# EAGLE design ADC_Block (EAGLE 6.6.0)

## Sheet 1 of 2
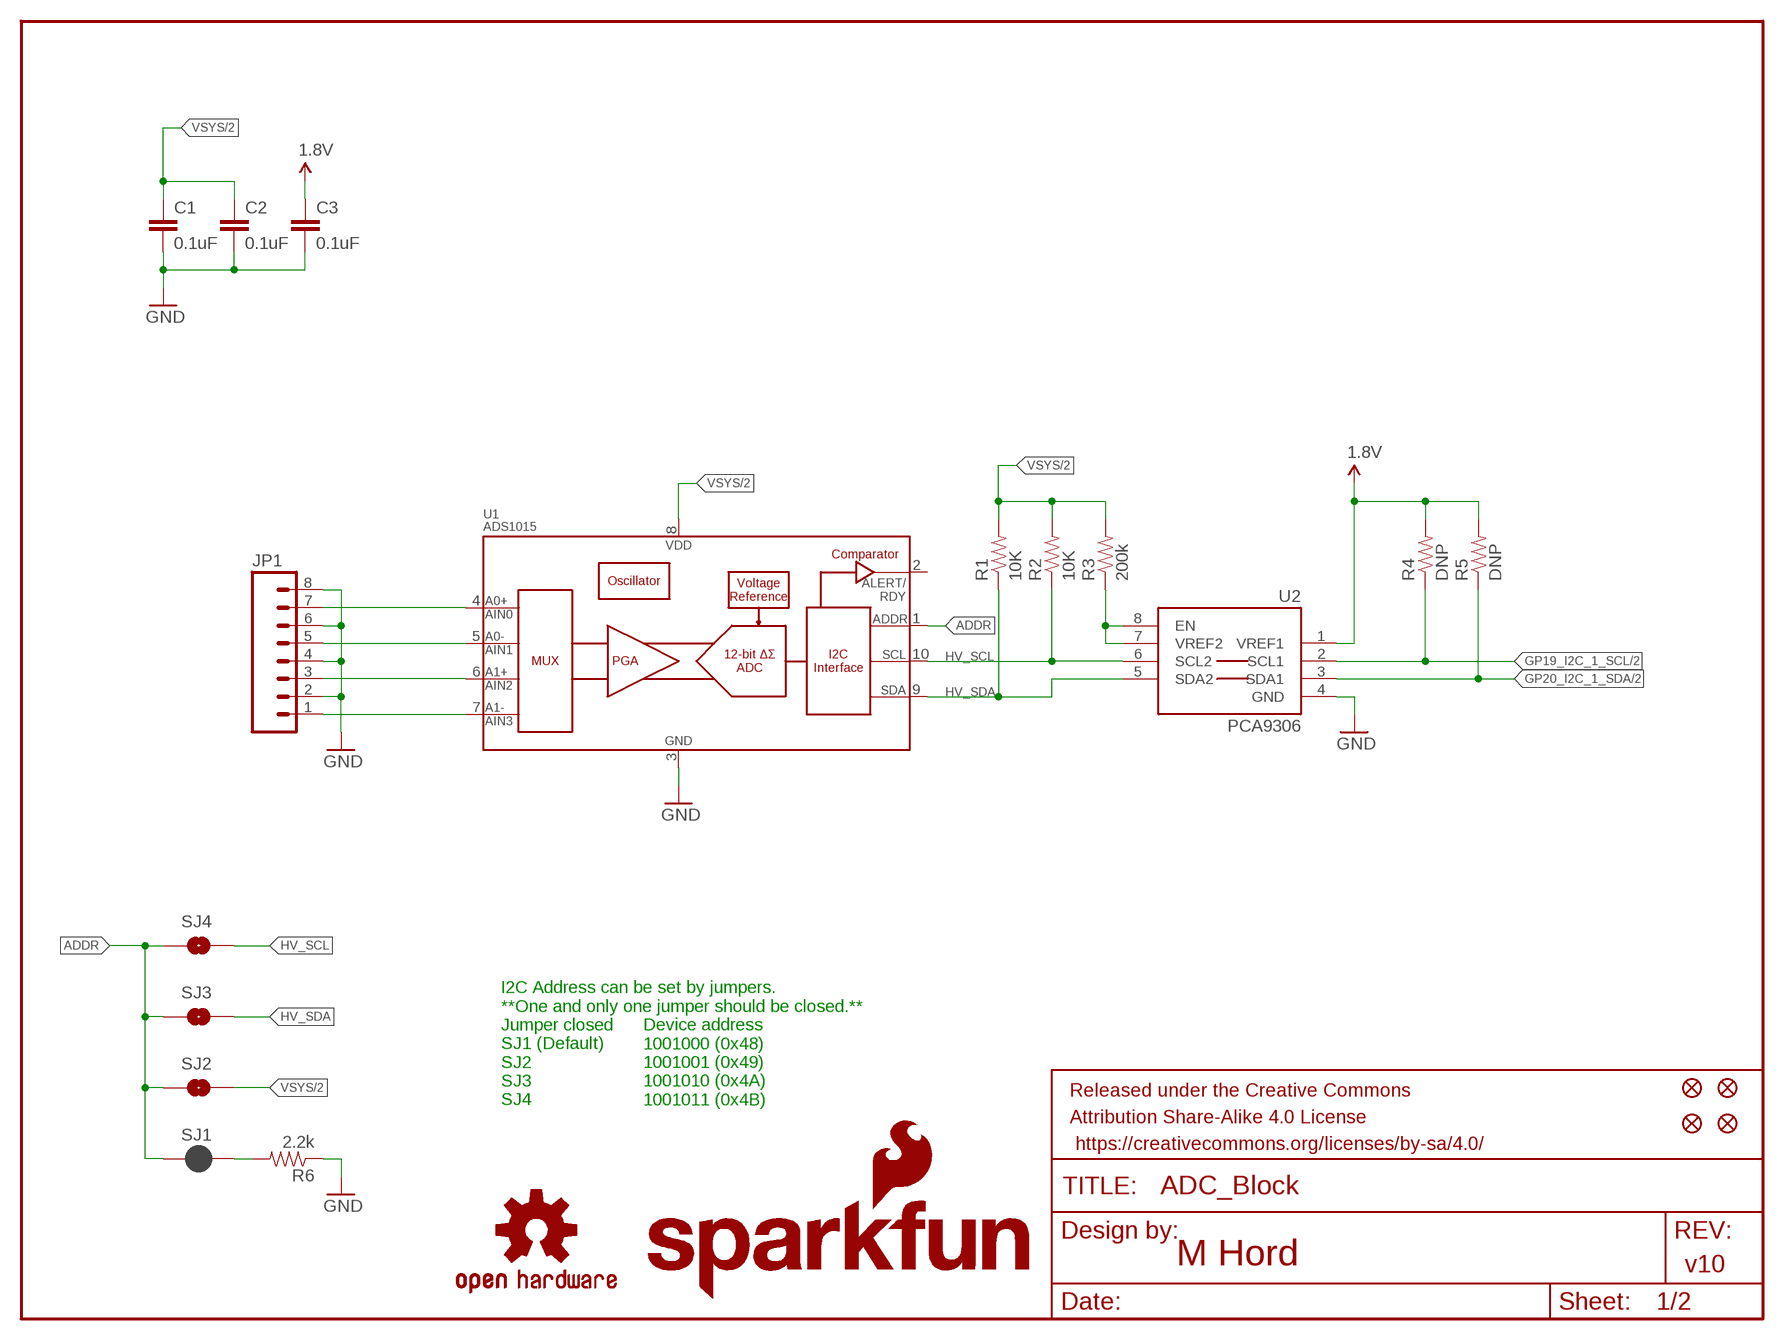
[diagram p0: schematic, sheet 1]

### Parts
C1  0.1uF  0.1UF-25V(+80/-20%)(0603)  [0603-CAP]
C2  0.1uF  0.1UF-25V(+80/-20%)(0603)  [0603-CAP]
C3  0.1uF  0.1UF-25V(+80/-20%)(0603)  [0603-CAP]
FID1  FIDUCIAL1X2  [FIDUCIAL-1X2]
FID2  FIDUCIAL1X2  [FIDUCIAL-1X2]
FID3  FIDUCIAL1X2  [FIDUCIAL-1X2]
FID4  FIDUCIAL1X2  [FIDUCIAL-1X2]
FRAME1  FRAME-LETTER  [CREATIVE_COMMONS]
JP1  M081X08  [1X08]
LOGO1  SFE_LOGO_NAME_FLAME.1_INCH  [SFE_LOGO_NAME_FLAME_.1]
LOGO2  OSHW-LOGOS  [OSHW-LOGO-S]
LOGO3  SFE_LOGO_NAME_FLAME.1_INCH  [SFE_LOGO_NAME_FLAME_.1]
LOGO4  OSHW-LOGOS  [OSHW-LOGO-S]
R1  10K  10KOHM1/10W1%(0603)0603  [0603-RES]
R2  10K  10KOHM1/10W1%(0603)0603  [0603-RES]
R3  200k  200KOHM1/10W1%(0603)200K  [0603-RES]
R4  DNP  2.2KOHM1/10W1%(0603)  [0603-RES]
R5  DNP  2.2KOHM1/10W1%(0603)  [0603-RES]
R6  2.2k  2.2KOHM1/10W1%(0603)  [0603-RES]
SJ1  JUMPER-PAD-2-NC_BY_PASTE  [PAD-JUMPER-2-NC_BY_PASTE_YES_SILK]
SJ2  JUMPER-PAD-2-NOYES_SILK  [PAD-JUMPER-2-NO_YES_SILK]
SJ3  JUMPER-PAD-2-NOYES_SILK  [PAD-JUMPER-2-NO_YES_SILK]
SJ4  JUMPER-PAD-2-NOYES_SILK  [PAD-JUMPER-2-NO_YES_SILK]
U1  ADS1015  [MSOP10]
U2  PCA9306  PCA9306PCA9306DC-1:1  [PCA9306DC-1:1]

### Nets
1.8V: C3.1 R4.2 R5.2 U2.1(VREF1) ; also sheet 2
A0+/AIN0: JP1.7 U1.4(AIN0)
A0-/AIN1: JP1.5 U1.5(AIN1)
A1+/AIN2: JP1.3 U1.6(AIN2)
A1-/AIN3: JP1.1 U1.7(AIN3)
ADDR: SJ1.1 SJ2.1 SJ3.1 SJ4.1 U1.1(ADDR)
GND: C1.2 C2.2 C3.2 JP1.2 JP1.4 JP1.6 JP1.8 R6.1 U1.3(VSS) U2.4(GND) ; also sheet 2
GP19_I2C_1_SCL: R4.1 U2.2(SCL1) ; also sheet 2
GP20_I2C_1_SDA: R5.1 U2.3(SDA1) ; also sheet 2
HV_SCL: R2.1 SJ4.2 U1.10(SCL) U2.6(SCL2)
HV_SDA: R1.1 SJ3.2 U1.9(SDA) U2.5(SDA2)
N$1: R3.1 U2.7(VREF2) U2.8(EN)
N$3: R6.2 SJ1.2
VSYS: C1.1 C2.1 R1.2 R2.2 R3.2 SJ2.2 U1.8(VDD) ; also sheet 2
Unconnected: U1.2(ALERT/RDY)

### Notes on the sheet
- I2C Address can be set by jumpers.
  **One and only one jumper should be closed.**
  Jumper closed
  SJ1 (Default)
  SJ2
  SJ3
  SJ4
- Device address
  1001000 (0x48)
  1001001 (0x49)
  1001010 (0x4A)
  1001011 (0x4B)
- M Hord
- v10

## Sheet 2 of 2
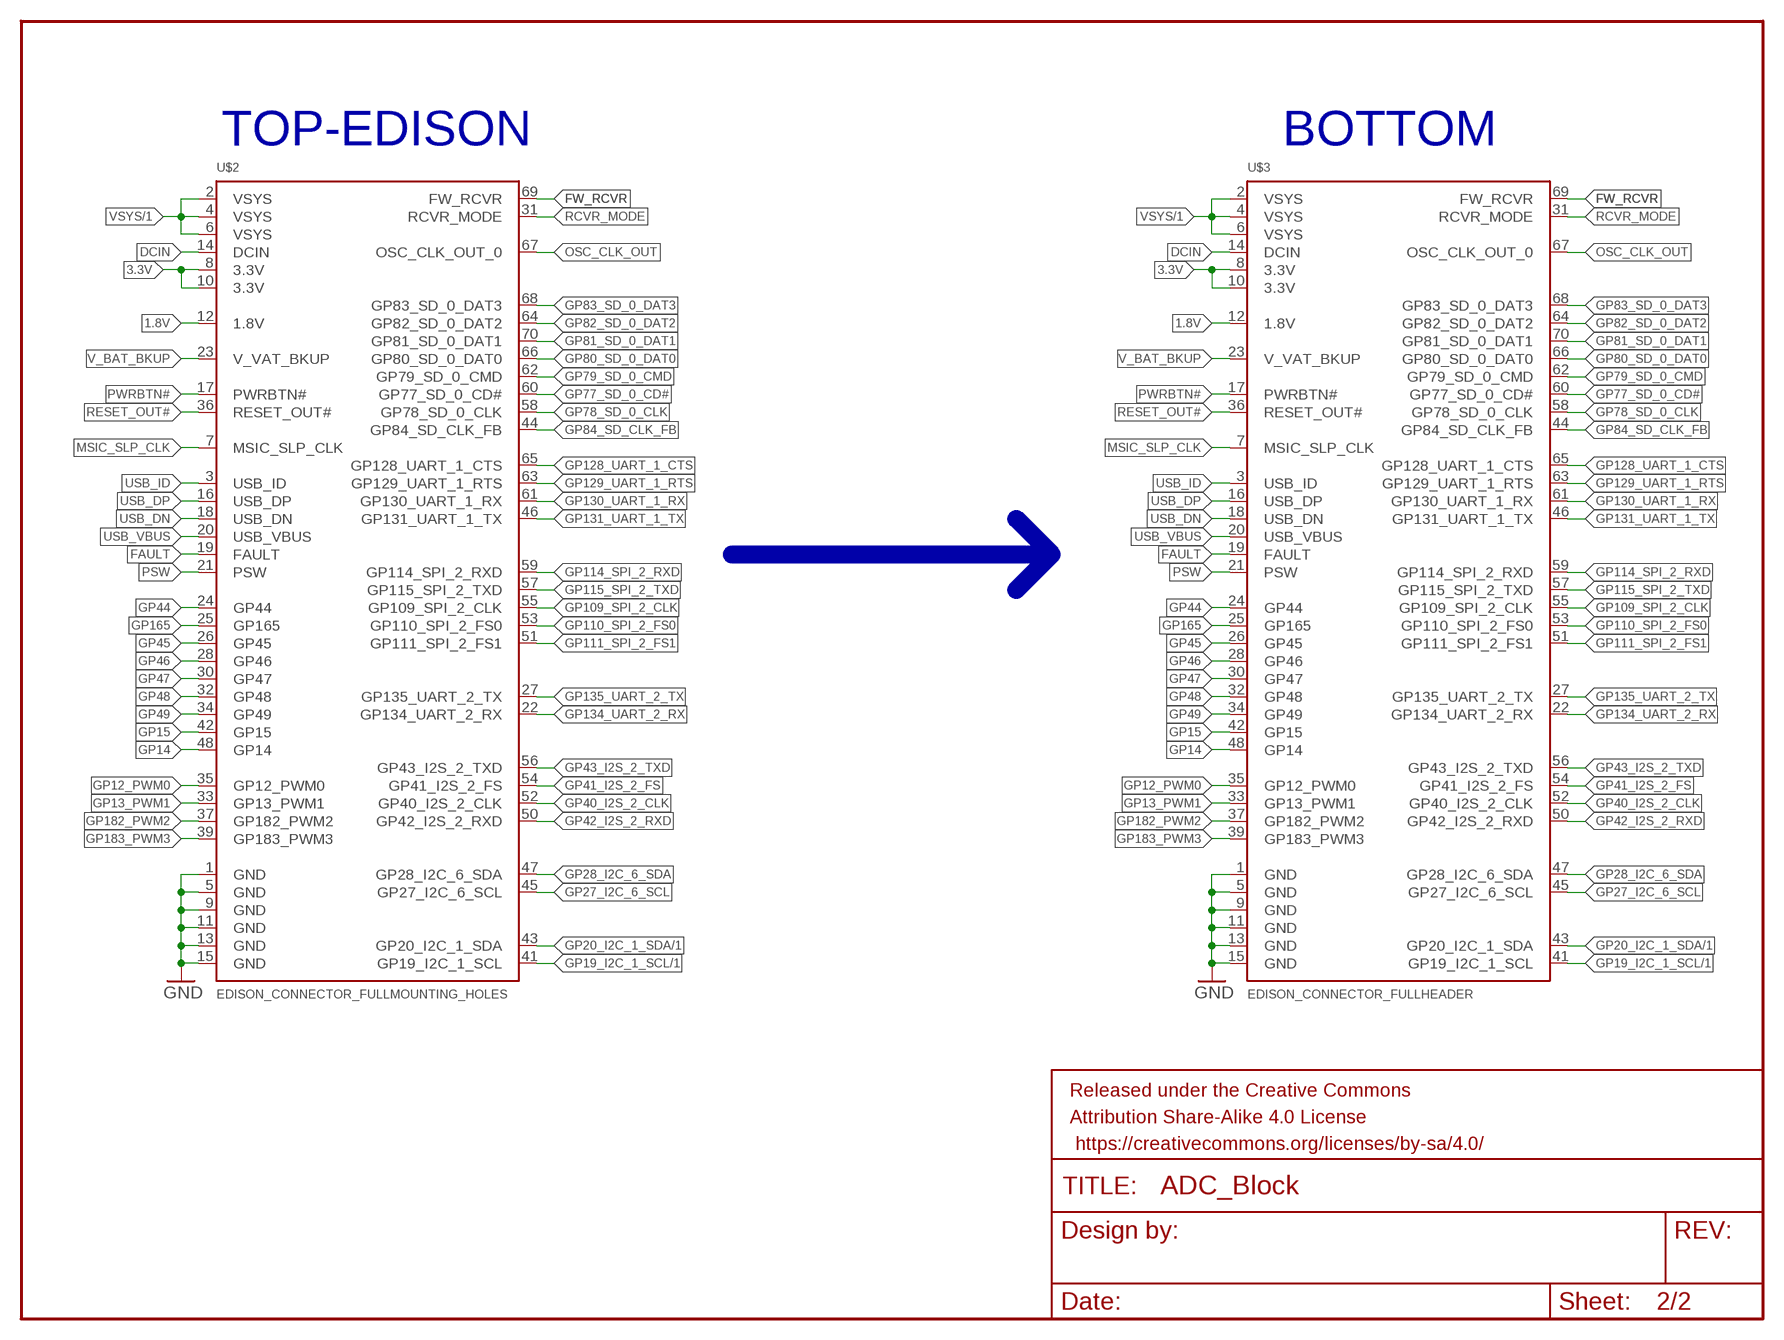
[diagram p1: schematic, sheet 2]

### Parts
FRAME2  FRAME-LETTER  [CREATIVE_COMMONS]
U$2  EDISON_CONNECTOR_FULLMOUNTING_HOLES  [EDISON_DAUGHTER]
U$3  EDISON_CONNECTOR_FULLHEADER  [DF40C-70DP-0.4(51)]

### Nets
1.8V: U$2.12(1.8V) U$3.12(1.8V) ; also sheet 1
3.3V: U$2.8(3.3V) U$2.10(3.3V) U$3.8(3.3V) U$3.10(3.3V)
DCIN: U$2.14(DCIN) U$3.14(DCIN)
FAULT: U$2.19(FAULT) U$3.19(FAULT)
FW_RCVR: U$2.69(FW_RCVR) U$3.69(FW_RCVR)
GND: U$2.1(GND) U$2.5(GND) U$2.9(GND) U$2.11(GND) U$2.13(GND) U$2.15(GND) U$3.1(GND) U$3.5(GND) U$3.9(GND) U$3.11(GND) U$3.13(GND) U$3.15(GND) ; also sheet 1
GP12_PWM0: U$2.35(GP12_PWM0) U$3.35(GP12_PWM0)
GP13_PWM1: U$2.33(GP13_PWM1) U$3.33(GP13_PWM1)
GP14: U$2.48(GP14) U$3.48(GP14)
GP15: U$2.42(GP15) U$3.42(GP15)
GP19_I2C_1_SCL: U$2.41(GP19_I2C_1_SCL) U$3.41(GP19_I2C_1_SCL) ; also sheet 1
GP20_I2C_1_SDA: U$2.43(GP20_I2C_1_SDA) U$3.43(GP20_I2C_1_SDA) ; also sheet 1
GP27_I2C_6_SCL: U$2.45(GP27_I2C_6_SCL) U$3.45(GP27_I2C_6_SCL)
GP28_I2C_6_SDA: U$2.47(GP28_I2C_6_SDA) U$3.47(GP28_I2C_6_SDA)
GP40_I2S_2_CLK: U$2.52(GP40_I2S_2_CLK) U$3.52(GP40_I2S_2_CLK)
GP41_I2S_2_FS: U$2.54(GP41_I2S_2_FS) U$3.54(GP41_I2S_2_FS)
GP42_I2S_2_RXD: U$2.50(GP42_I2S_2_RXD) U$3.50(GP42_I2S_2_RXD)
GP43_I2S_2_TXD: U$2.56(GP43_I2S_2_TXD) U$3.56(GP43_I2S_2_TXD)
GP44: U$2.24(GP44) U$3.24(GP44)
GP45: U$2.26(GP45) U$3.26(GP45)
GP46: U$2.28(GP46) U$3.28(GP46)
GP47: U$2.30(GP47) U$3.30(GP47)
GP48: U$2.32(GP48) U$3.32(GP48)
GP49: U$2.34(GP49) U$3.34(GP49)
GP77_SD_0_CD#: U$2.60(GP77_SD_0_CD#) U$3.60(GP77_SD_0_CD#)
GP78_SD_0_CLK: U$2.58(GP78_SD_0_CLK) U$3.58(GP78_SD_0_CLK)
GP79_SD_0_CMD: U$2.62(GP79_SD_0_CMD) U$3.62(GP79_SD_0_CMD)
GP80_SD_0_DAT0: U$2.66(GP80_SD_0_DAT0) U$3.66(GP80_SD_0_DAT0)
GP81_SD_0_DAT1: U$2.70(GP81_SD_0_DAT1) U$3.70(GP81_SD_0_DAT1)
GP82_SD_0_DAT2: U$2.64(GP82_SD_0_DAT2) U$3.64(GP82_SD_0_DAT2)
GP83_SD_0_DAT3: U$2.68(GP83_SD_0_DAT3) U$3.68(GP83_SD_0_DAT3)
GP84_SD_CLK_FB: U$2.44(GP84_SD_CLK_FB) U$3.44(GP84_SD_CLK_FB)
GP109_SPI_2_CLK: U$2.55(GP109_SPI_2_CLK) U$3.55(GP109_SPI_2_CLK)
GP110_SPI_2_FS0: U$2.53(GP110_SPI_2_FS0) U$3.53(GP110_SPI_2_FS0)
GP111_SPI_2_FS1: U$2.51(GP111_SPI_2_FS1) U$3.51(GP111_SPI_2_FS1)
GP114_SPI_2_RXD: U$2.59(GP114_SPI_2_RXD) U$3.59(GP114_SPI_2_RXD)
GP115_SPI_2_TXD: U$2.57(GP115_SPI_2_TXD) U$3.57(GP115_SPI_2_TXD)
GP128_UART_1_CTS: U$2.65(GP128_UART_1_CTS) U$3.65(GP128_UART_1_CTS)
GP129_UART_1_RTS: U$2.63(GP129_UART_1_RTS) U$3.63(GP129_UART_1_RTS)
GP130_UART_1_RX: U$2.61(GP130_UART_1_RX) U$3.61(GP130_UART_1_RX)
GP131_UART_1_TX: U$2.46(GP131_UART_1_TX) U$3.46(GP131_UART_1_TX)
GP134_UART_2_RX: U$2.22(GP134_UART_2_RX) U$3.22(GP134_UART_2_RX)
GP135_UART_2_TX: U$2.27(GP135_UART_2_TX) U$3.27(GP135_UART_2_TX)
GP165: U$2.25(GP165) U$3.25(GP165)
GP182_PWM2: U$2.37(GP182_PWM2) U$3.37(GP182_PWM2)
GP183_PWM3: U$2.39(GP183_PWM3) U$3.39(GP183_PWM3)
MSIC_SLP_CLK: U$2.7(MSIC_SLP_CLK) U$3.7(MSIC_SLP_CLK)
OSC_CLK_OUT: U$2.67(OSC_CLK_OUT_0) U$3.67(OSC_CLK_OUT_0)
PSW: U$2.21(PSW) U$3.21(PSW)
PWRBTN#: U$2.17(PWRBTN#) U$3.17(PWRBTN#)
RCVR_MODE: U$2.31(RCVR_MODE) U$3.31(RCVR_MODE)
RESET_OUT#: U$2.36(RESET_OUT#) U$3.36(RESET_OUT#)
USB_DN: U$2.18(USB_DN) U$3.18(USB_DN)
USB_DP: U$2.16(USB_DP) U$3.16(USB_DP)
USB_ID: U$2.3(USB_ID) U$3.3(USB_ID)
USB_VBUS: U$2.20(USB_VBUS) U$3.20(USB_VBUS)
V_BAT_BKUP: U$2.23(V_VAT_BKUP) U$3.23(V_VAT_BKUP)
VSYS: U$2.2(VSYS) U$2.4(VSYS) U$2.6(VSYS) U$3.2(VSYS) U$3.4(VSYS) U$3.6(VSYS) ; also sheet 1

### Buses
B$1

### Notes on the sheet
- TOP-EDISON | BOTTOM

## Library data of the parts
C1-C3 = SparkFun-Capacitors:0.1UF-25V(+80/-20%)(0603): CAP-00810; PROD_ID: CAP-00810
FID1-FID4 = SparkFun-Aesthetics:FIDUCIAL: Fiducial Alignment Points
FRAME1 FRAME2 = SparkFun-Aesthetics:FRAME-LETTER: Schematic Frame
JP1 = SparkFun-Connectors:M08: Header 8 Standard 8-pin 0.1" header. Use with straight break away headers (SKU : PRT-00116), right angle break away headers (PRT-00553), swiss pins (PRT-00743), machine pins (PRT-00117), and female headers (PRT-00115).
LOGO1 LOGO3 = SparkFun-Aesthetics:SFE_LOGO_NAME_FLAME: SFE Logo, name and flame
LOGO2 LOGO4 = SparkFun-Aesthetics:OSHW-LOGO: Open Source Hardware Logo This logo indicates the piece of hardware it is found on incorporates a OSHW license and/or adheres to the definition of open source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
R1 R2 = SparkFun-Resistors:10KOHM1/10W1%(0603): RES-00824; PROD_ID: RES-00824
R3 = SparkFun-Resistors:200KOHM1/10W1%(0603): RES-09385; PROD_ID: RES-09385
R4 R5 = SparkFun-Resistors:2.2KOHM1/10W1%(0603): RES-08272; PROD_ID: RES-08272; VALUE: 2.2k
R6 = SparkFun-Resistors:2.2KOHM1/10W1%(0603): RES-08272; PROD_ID: RES-08272
SJ1 = SparkFun-Passives:JUMPER-PAD-2-NC_BY_PASTE
SJ2-SJ4 = SparkFun-Passives:JUMPER-PAD-2-NO
U1 = SparkFun-AnalogIC:ADS1015: 12-Bit Del-Sig ADC Four single-ended inputs or two differential inputs Internal PGA I2C interface 2.0-5.5V; PROD_ID: IC-12239
U2 = SparkFun-DigitalIC:PCA9306: Bidirectional I2C level shifter. NOT compatible with all available part number pinout schemes- DOUBLE CHECK!!!; PROD_ID: IC-10023
U$2 U$3 = Edison:EDISON_CONNECTOR_FULL

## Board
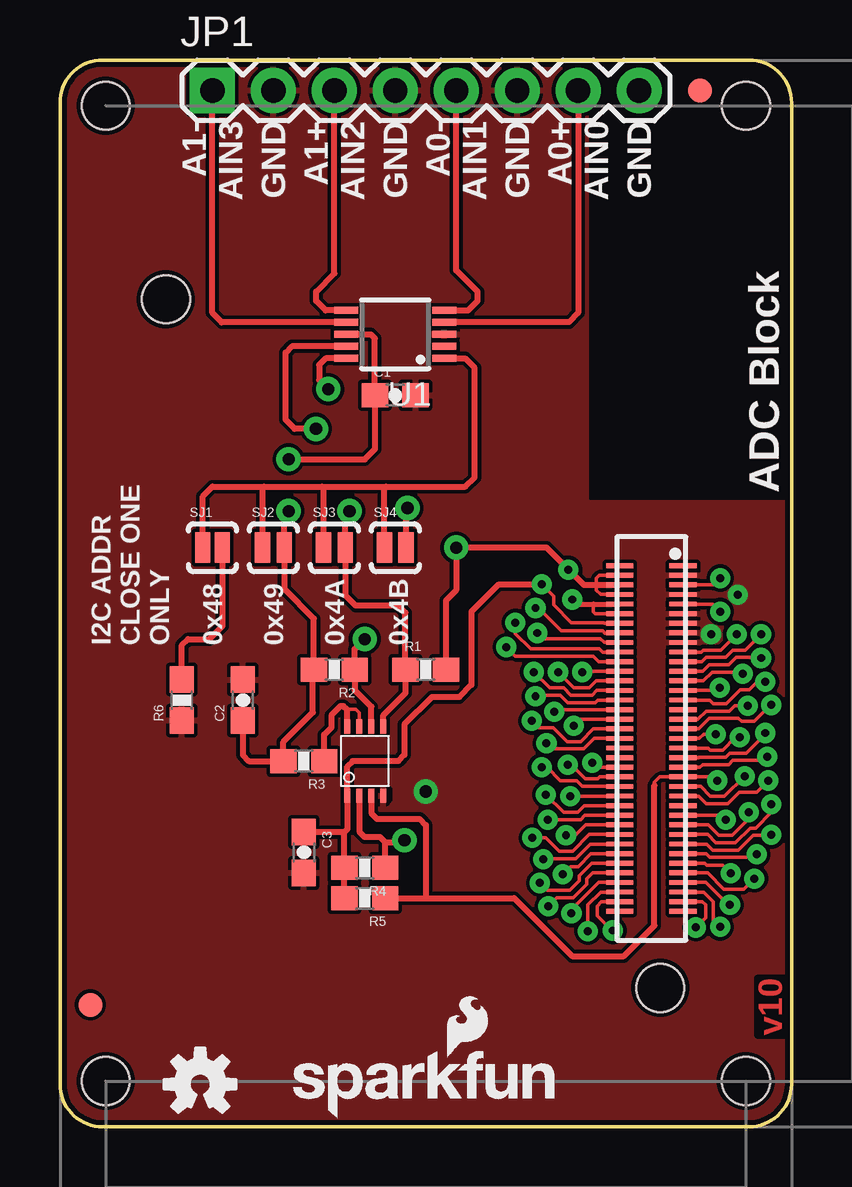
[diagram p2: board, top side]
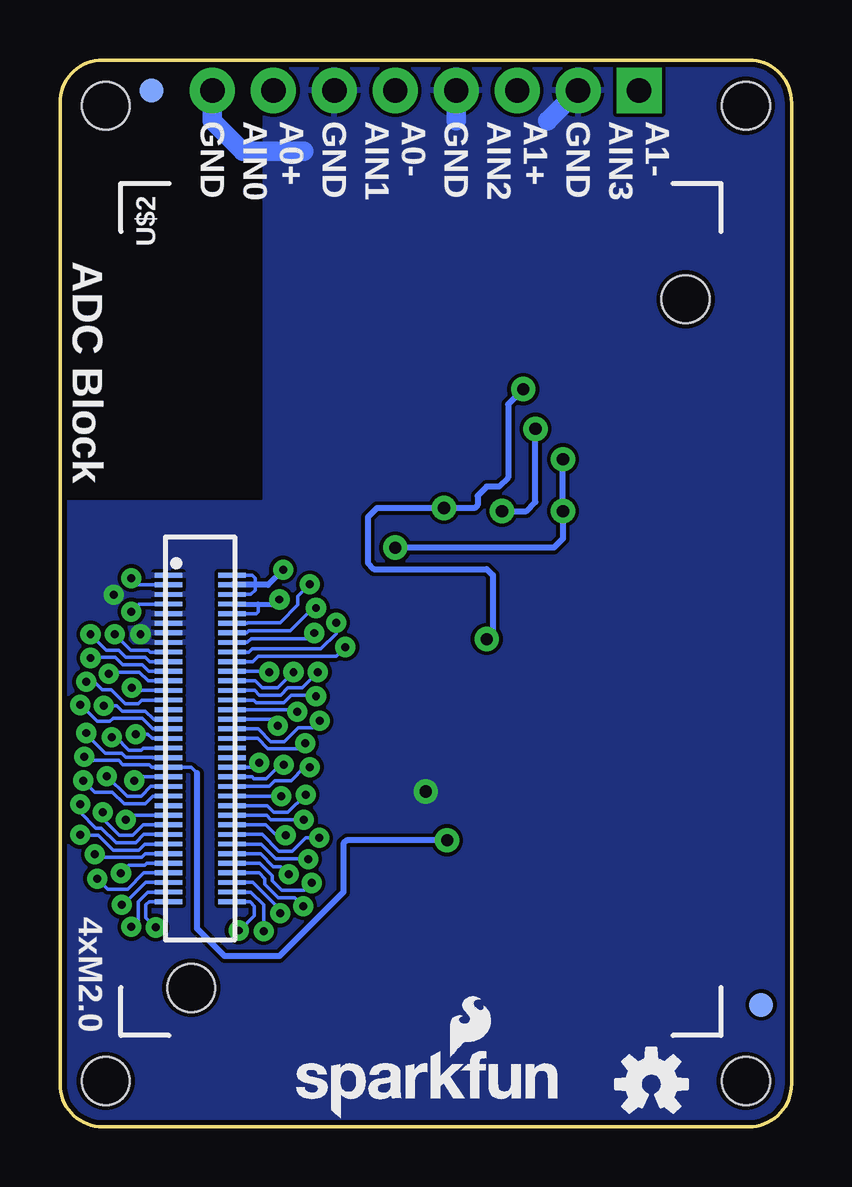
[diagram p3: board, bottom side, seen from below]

Size 30.48 x 44.45 mm. Coordinates in mm from the lower left corner, seen from the top.
Outline: 30.48,42.67 30.48,1.78 arc-90 28.7,0 1.78,0 arc-90 0,1.78 0,42.67 arc-90 1.78,44.45 28.7,44.45 arc-90 30.48,42.67
Copper layers (1*16): Top 0.035mm / dielectric 1.5mm / Bottom 0.035mm
Design rules "SparkFun-2-layer *": minimum track width 6mil, minimum drill 13mil, track to track 6mil, track to pad 6mil, pad to pad 6mil, via to via 6mil, smd to smd 6mil, copper to edge 8mil, drill to drill 8mil, minimum pad ring 12mil, minimum via ring 10mil, stop-mask expansion 4mil, vias tented up to drill 20mil, thermal gap 6mil
Holes 2 mm at 28.57,1.91 1.91,1.91 1.91,42.55 28.57,42.55
tRestrict: area 22.1,26.2 to 30.5,44.5; 1 lines
bRestrict: area 22.1,26.2 to 30.5,44.5

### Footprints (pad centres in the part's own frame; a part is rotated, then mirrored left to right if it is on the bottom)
0603-CAP = smd 1.1 x 1: 1 -0.85,0; 2 0.85,0
FIDUCIAL-1X2 = smd 1 x 1: 1 0,0
1X08 = drill 1.016 pad 1.88 square: 1 0,0 | drill 1.016 pad 1.88: 2 2.54,0; 3 5.08,0; 4 7.62,0; 5 10.16,0; 6 12.7,0; 7 15.24,0; 8 17.78,0
0603-RES = smd 1.1 x 1: 1 -0.85,0; 2 0.85,0
PAD-JUMPER-2-NC_BY_PASTE_YES_SILK = smd 0.635 x 1.27: 1 -0.401,0; 2 0.413,0
PAD-JUMPER-2-NO_YES_SILK = smd 0.635 x 1.27: 1 -0.45,0; 2 0.45,0
MSOP10 = smd 0.3 x 1: 1 -1,-2.05; 2 -0.5,-2.05; 3 0,-2.05; 4 0.5,-2.05; 5 1,-2.05; 6 1,2.05; 7 0.5,2.05; 8 0,2.05; 9 -0.5,2.05; 10 -1,2.05
PCA9306DC-1:1 = smd 0.25 x 0.602: 1 -0.73,-1.446; 2 -0.23,-1.446; 3 0.27,-1.446; 4 0.77,-1.446; 5 0.77,1.431; 6 0.27,1.431; 7 -0.23,1.431; 8 -0.73,1.431
EDISON_DAUGHTER = smd 1.14 x 0.2: 1 1.98,19.17; 2 4.62,19.17; 3 1.98,18.77; 4 4.62,18.77; 5 1.98,18.37; 6 4.62,18.37; 7 1.98,17.97; 8 4.62,17.97; 9 1.98,17.57; 10 4.62,17.57; 11 1.98,17.17; 12 4.62,17.17; 13 1.98,16.77; 14 4.62,16.77; 15 1.98,16.37; 16 4.62,16.37; 17 1.98,15.97; 18 4.62,15.97; 19 1.98,15.57; 20 4.62,15.57; 21 1.98,15.17; 22 4.62,15.17; 23 1.98,14.77; 24 4.62,14.77; 25 1.98,14.37; 26 4.62,14.37; 27 1.98,13.97; 28 4.62,13.97; 29 1.98,13.57; 30 4.62,13.57; 31 1.98,13.17; 32 4.62,13.17; 33 1.98,12.77; 34 4.62,12.77; 35 1.98,12.37; 36 4.62,12.37; 37 1.98,11.97; 38 4.62,11.97; 39 1.98,11.57; 40 4.62,11.57; 41 1.98,11.17; 42 4.62,11.17; 43 1.98,10.77; 44 4.62,10.77; 45 1.98,10.37; 46 4.62,10.37; 47 1.98,9.97; 48 4.62,9.97; 49 1.98,9.57; 50 4.62,9.57; 51 1.98,9.17; 52 4.62,9.17; 53 1.98,8.77; 54 4.62,8.77; 55 1.98,8.37; 56 4.62,8.37; 57 1.98,7.97; 58 4.62,7.97; 59 1.98,7.57; 60 4.62,7.57; 61 1.98,7.17; 62 4.62,7.17; 63 1.98,6.77; 64 4.62,6.77; 65 1.98,6.37; 66 4.62,6.37; 67 1.98,5.97; 68 4.62,5.97; 69 1.98,5.57; 70 4.62,5.57 | hole 2: 23.53,30.67; 2.93,1.98
DF40C-70DP-0.4(51) = smd 0.2 x 1.14 bottom: 1 6.8,1.32; 2 6.8,-1.32; 3 6.4,1.32; 4 6.4,-1.32; 5 6,1.32; 6 6,-1.32; 7 5.6,1.32; 8 5.6,-1.32; 9 5.2,1.32; 10 5.2,-1.32; 11 4.8,1.32; 12 4.8,-1.32; 13 4.4,1.32; 14 4.4,-1.32; 15 4,1.32; 16 4,-1.32; 17 3.6,1.32; 18 3.6,-1.32; 19 3.2,1.32; 20 3.2,-1.32; 21 2.8,1.32; 22 2.8,-1.32; 23 2.4,1.32; 24 2.4,-1.32; 25 2,1.32; 26 2,-1.32; 27 1.6,1.32; 28 1.6,-1.32; 29 1.2,1.32; 30 1.2,-1.32; 31 0.8,1.32; 32 0.8,-1.32; 33 0.4,1.32; 34 0.4,-1.32; 35 0,1.32; 36 0,-1.32; 37 -0.4,1.32; 38 -0.4,-1.32; 39 -0.8,1.32; 40 -0.8,-1.32; 41 -1.2,1.32; 42 -1.2,-1.32; 43 -1.6,1.32; 44 -1.6,-1.32; 45 -2,1.32; 46 -2,-1.32; 47 -2.4,1.32; 48 -2.4,-1.32; 49 -2.8,1.32; 50 -2.8,-1.32; 51 -3.2,1.32; 52 -3.2,-1.32; 53 -3.6,1.32; 54 -3.6,-1.32; 55 -4,1.32; 56 -4,-1.32; 57 -4.4,1.32; 58 -4.4,-1.32; 59 -4.8,1.32; 60 -4.8,-1.32; 61 -5.2,1.32; 62 -5.2,-1.32; 63 -5.6,1.32; 64 -5.6,-1.32; 65 -6,1.32; 66 -6,-1.32; 67 -6.4,1.32; 68 -6.4,-1.32; 69 -6.8,1.32; 70 -6.8,-1.32; NC1 7.2,1.32; NC2 7.2,-1.32; NC3 -7.2,-1.32; NC4 -7.2,1.32

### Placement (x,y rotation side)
C1  13.97,30.48 0 top
C2  7.62,17.78 90 top
C3  10.16,11.43 270 top
FID1  1.27,5.08 0 top
FID2  26.67,43.18 0 top
FID3  26.67,43.18 0 bottom
FID4  1.27,5.08 0 bottom
FRAME1  not placed on the board
FRAME2  not placed on the board
JP1  6.35,43.18 0 top
LOGO1  9.27,0.25 0 top
LOGO2  5.84,1.78 0 bottom
LOGO3  21.08,0.25 0 bottom
LOGO4  5.84,1.78 0 top
R1  15.24,19.05 0 top
R2  11.43,19.05 180 top
R3  10.16,15.24 180 top
R4  12.7,10.79 180 top
R5  12.7,9.53 180 top
R6  5.08,17.78 90 top
SJ1  6.35,24.13 0 top
SJ2  8.89,24.13 0 top
SJ3  11.43,24.13 0 top
SJ4  13.97,24.13 0 top
U1  13.97,33.02 90 top
U2  12.7,15.24 0 top
U$2  27.94,3.81 0 bottom
U$3  24.64,16.18 90 bottom

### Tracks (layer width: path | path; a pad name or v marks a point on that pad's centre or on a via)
1.8V  (via drill 0.33)
  Top 0.152: U$3.12 22.68,20.98 22.66,21.01 21.31,21.01 20.57,21.74 20.57,22.1 v20.07,22.61
  Top 0.254: R5.2 R4.2 11.85,12.28 | 11.85,12.28 11.97,12.4 U2.1 11.97,15.02 12.19,15.24 14.1,15.24 14.35,15.49 14.35,16.76 15.49,17.91 16.64,17.91 17.14,18.41 17.14,21.46 18.29,22.61 v20.07,22.61 | 11.85,12.28 C3.1
  Bottom 0.152: v20.07,22.61 20.57,22.1 20.57,21.74 21.31,21.01 22.66,21.01 22.68,20.98 U$3.12
3.3V  (via drill 0.33)
  Top 0.152: U$3.10 22.31,21.38 22.23,21.46 22.23,21.78
  Top 0.203: v21.34,21.97 21.53,21.78 22.23,21.78 U$3.8
  Bottom 0.152: U$3.10 22.31,21.38 22.23,21.46 22.23,21.78 | U$3.8
  Bottom 0.203: U$3.8 22.23,21.78 21.53,21.78 v21.34,21.97
A0+/AIN0
  Top 0.254: JP1.7 21.59,33.91 21.21,33.53 U1.4
A0-/AIN1
  Top 0.254: U1.5 17,34.02 17.4,34.42 17.4,34.8 16.51,35.69 JP1.5
A1+/AIN2
  Top 0.254: U1.6 11.06,34.02 10.67,34.42 10.67,34.8 11.43,35.56 JP1.3
A1-/AIN3
  Top 0.254: U1.7 6.74,33.52 6.35,33.91 JP1.1
ADDR
  Top 0.254: SJ1.1 5.95,26.27 6.35,26.67 8.51,26.67 | 8.51,26.67 10.92,26.67 | 10.92,26.67 13.59,26.67 | 13.59,26.67 16.89,26.67 17.27,27.05 17.27,31.62 16.88,32.02 U1.1 | SJ2.1 8.44,26.6 8.51,26.67 | SJ3.1 10.98,26.61 10.92,26.67 | SJ4.1 13.52,26.6 13.59,26.67
DCIN  (via drill 0.33)
  Top 0.152: v19.81,21.61 19.94,21.61 20.88,20.68 22.61,20.68 22.71,20.57 U$2.14
  Bottom 0.152: U$2.14 22.7,20.58 22.61,20.68 20.88,20.68 19.94,21.61 v19.81,21.61
FAULT  (via drill 0.33)
  Top 0.152: U$3.19 26.75,19.38 26.92,19.56 27.74,19.56 28.04,19.86 28.55,19.86 v29.21,20.52
  Bottom 0.152: v29.21,20.52 28.55,19.86 28.04,19.86 27.74,19.56 26.92,19.56 26.75,19.38 U$3.19
FW_RCVR  (via drill 0.33)
  Top 0.152: v26.49,8.31 26.9,8.71 26.9,9.25 26.76,9.38 U$3.69
  Bottom 0.152: U$3.69 26.76,9.38 26.9,9.25 26.9,8.71 v26.49,8.31
GND  (via drill 0.33, 0.51)
  Bottom 0.813: JP1.2 10.16,41.91 | JP1.4 13.97,41.91 | JP1.8 24.13,41.91 22.86,40.64 20.32,40.64
  other vias: 27.13,20.52 28.24,22.17 15.24,13.97
  pour Bottom (isolate 0.051, rank 6): 30.48,42.67 30.48,1.78 arc-90 28.7,0 1.78,0 arc-90 0,1.78 0,42.67 arc-90 1.78,44.45 28.7,44.45 arc-90
  pour Top (isolate 0.051, rank 6): 30.48,1.73 arc-90 28.75,0 1.78,0 arc-90 0,1.78 0,42.67 arc-90 1.78,44.45 28.7,44.45 arc-90 30.48,42.67
GP12_PWM0  (via drill 0.33)
  Top 0.152: U$3.35 26.64,16.18 26.82,16.36 v27.33,16.36
  Bottom 0.152: v27.33,16.36 26.82,16.36 26.64,16.18 U$3.35 | U$3.35
GP13_PWM1  (via drill 0.33)
  Top 0.152: v29.64,17.58 29.62,17.58 28.93,16.89 28.4,16.89 28.27,17.02 27.05,17.02 26.61,16.58 U$3.33
  Bottom 0.152: U$3.33 26.61,16.58 27.05,17.02 28.27,17.02 28.4,16.89 28.93,16.89 29.62,17.58 v29.64,17.58
GP14  (via drill 0.33)
  Top 0.152: v21.26,13.77 21.27,13.78 U$3.48
  Bottom 0.152: U$3.48 21.27,13.78 v21.26,13.77
GP15  (via drill 0.33)
  Top 0.152: U$3.42 22.36,14.98 v22.17,15.16
  Bottom 0.152: v22.17,15.16 22.36,14.98 U$3.42
GP19_I2C_1_SCL  (via drill 0.33, 0.51)
  Top 0.152: U$3.41 26.66,14.98 26.77,15.09 27.86,15.09 28.04,15.27 29.31,15.27 v29.46,15.42
  Top 0.254: U2.2 12.47,12.29 12.7,12.06 13.34,12.06 13.55,11.85 | R4.1 13.55,11.85 | 13.55,11.85 14.26,11.85 v14.35,11.94
  Bottom 0.152: v29.46,15.42 29.31,15.27 28.04,15.27 27.86,15.09 26.77,15.09 26.66,14.98 U$3.41 25.01,14.98 24.77,14.73
  Bottom 0.254: v14.35,11.94 18.54,11.94 18.67,11.81 18.67,9.78 21.34,7.11 23.62,7.11 24.77,8.26 24.77,14.73
GP20_I2C_1_SDA  (via drill 0.33)
  Top 0.152: v27.38,14.43 27.23,14.58 U$3.43 24.99,14.58 24.77,14.35 24.77,14.22
  Top 0.254: U2.3 12.97,13.06 13.21,12.83 14.99,12.83 15.24,12.57 15.24,9.53 | R5.1 15.24,9.53 | 15.24,9.53 18.92,9.53 21.34,7.11 23.5,7.11 24.77,8.38 24.77,14.22
  Bottom 0.152: v27.38,14.43 27.23,14.58 U$3.43 | U$3.43
GP27_I2C_6_SCL  (via drill 0.33)
  Top 0.152: v28.52,14.61 27.69,13.77 27.1,13.77 26.69,14.18 U$3.45
  Bottom 0.152: U$3.45 26.69,14.18 27.1,13.77 27.69,13.77 v28.52,14.61
GP28_I2C_6_SDA  (via drill 0.33)
  Top 0.152: U$3.47 26.61,13.78 26.92,13.46 27.81,13.46 28.3,13.95 29.03,13.95 v29.52,14.43
  Bottom 0.152: v29.52,14.43 29.03,13.95 28.3,13.95 27.81,13.46 26.92,13.46 26.61,13.78 U$3.47
GP40_I2S_2_CLK  (via drill 0.33)
  Top 0.152: U$3.52 21.87,12.98 21.69,12.8 v20.32,12.8
  Bottom 0.152: v20.32,12.8 21.69,12.8 21.87,12.98 U$3.52
GP41_I2S_2_FS  (via drill 0.33)
  Top 0.152: v21.08,12.14 21.46,12.14 21.9,12.58 U$3.54
  Bottom 0.152: U$3.54 21.9,12.58 21.46,12.14 v21.08,12.14
GP42_I2S_2_RXD  (via drill 0.33)
  Top 0.152: U$3.50 21.84,13.38 21.57,13.11 20.98,13.11 v20.24,13.84
  Bottom 0.152: v20.24,13.84 20.98,13.11 21.57,13.11 21.84,13.38 U$3.50
GP43_I2S_2_TXD  (via drill 0.33)
  Top 0.152: U$3.56 22.06,12.18 21.36,11.48 20.8,11.48 20.24,12.04 v19.68,12.04
  Bottom 0.152: v19.68,12.04 20.24,12.04 20.8,11.48 21.36,11.48 22.06,12.18 U$3.56
GP44  (via drill 0.33)
  Top 0.152: U$3.24 22.34,18.58 22.05,18.29 21.41,18.29 v20.75,18.95
  Bottom 0.152: v20.75,18.95 21.41,18.29 22.05,18.29 22.34,18.58 U$3.24
GP45  (via drill 0.33)
  Top 0.152: v19.74,18.95 20.4,18.29 20.98,18.29 21.29,17.98 22.17,17.98 22.37,18.18 U$3.26
  Bottom 0.152: U$3.26 22.37,18.18 22.17,17.98 21.29,17.98 20.98,18.29 20.4,18.29 v19.74,18.95
GP46  (via drill 0.33)
  Top 0.152: U$3.28 22.4,17.78 22.3,17.68 21.16,17.68 20.85,17.98 19.86,17.98 v19.81,17.93
  Bottom 0.152: v19.81,17.93 19.86,17.98 20.85,17.98 21.16,17.68 22.3,17.68 22.4,17.78 U$3.28
GP47  (via drill 0.33)
  Top 0.152: U$3.30 22.43,17.38 22.43,17.37 20.68,17.37 v20.6,17.3
  Bottom 0.152: v20.6,17.3 20.68,17.37 22.43,17.37 22.43,17.38 U$3.30
GP48  (via drill 0.33)
  Top 0.152: v21.41,16.71 21.68,16.98 U$3.32
  Bottom 0.152: U$3.32 21.68,16.98 v21.41,16.71
GP49  (via drill 0.33)
  Top 0.152: U$3.34 22.22,16.58 21.69,16.05 21.13,16.05 20.55,16.64 19.94,16.64 v19.66,16.92
  Bottom 0.152: v19.66,16.92 19.94,16.64 20.55,16.64 21.13,16.05 21.69,16.05 22.22,16.58 U$3.34
GP77_SD_0_CD#  (via drill 0.33)
  Top 0.152: U$3.60 22.12,11.38 21.59,10.85 21.29,10.85 v20.95,10.52
  Bottom 0.152: v20.95,10.52 21.29,10.85 21.59,10.85 22.12,11.38 U$3.60
GP78_SD_0_CLK  (via drill 0.33)
  Top 0.152: U$3.58 22.09,11.78 21.49,11.18 20.17,11.18 v20.14,11.15
  Bottom 0.152: v20.14,11.15 20.17,11.18 21.49,11.18 22.09,11.78 U$3.58
GP79_SD_0_CMD  (via drill 0.33)
  Top 0.152: U$3.62 22.16,10.98 21.64,10.46 21.64,10.26 21.23,9.86 20.3,9.86 v19.99,10.16
  Bottom 0.152: v19.99,10.16 20.3,9.86 21.23,9.86 21.64,10.26 21.64,10.46 22.16,10.98 U$3.62
GP80_SD_0_DAT0  (via drill 0.33)
  Top 0.152: v21.31,8.89 21.31,9.04 22.45,10.18 U$3.66
  Bottom 0.152: U$3.66 22.45,10.18 21.31,9.04 v21.31,8.89
GP81_SD_0_DAT1  (via drill 0.33)
  Top 0.152: U$3.70 22.56,9.38 22.38,9.2 22.38,8.79 22.99,8.18 v23.04,8.18
  Bottom 0.152: v23.04,8.18 22.99,8.18 22.38,8.79 22.38,9.2 22.56,9.38 U$3.70
GP82_SD_0_DAT2  (via drill 0.33)
  Top 0.152: U$3.64 22.19,10.58 21.95,10.34 21.95,10.11 21.39,9.55 20.7,9.55 v20.34,9.2
  Bottom 0.152: v20.34,9.2 20.7,9.55 21.39,9.55 21.95,10.11 21.95,10.34 22.19,10.58 U$3.64
GP83_SD_0_DAT3  (via drill 0.33)
  Top 0.152: v22,8.15 22,9.25 22.53,9.78 U$3.68
  Bottom 0.152: U$3.68 22.53,9.78 22,9.25 v22,8.15
GP84_SD_CLK_FB  (via drill 0.33)
  Top 0.152: U$3.44 22.48,14.58 22.4,14.5 21.89,14.5 21.31,15.09 v21.16,15.09
  Bottom 0.152: v21.16,15.09 21.31,15.09 21.89,14.5 22.4,14.5 22.48,14.58 U$3.44 | U$3.44
GP109_SPI_2_CLK  (via drill 0.33)
  Top 0.152: U$3.55 26.99,12.18 27.33,11.84 28.14,11.84 28.75,12.45 28.98,12.45 29.64,13.11 v29.64,13.44
  Bottom 0.152: v29.64,13.44 29.64,13.11 28.98,12.45 28.75,12.45 28.14,11.84 27.33,11.84 26.99,12.18 U$3.55
GP110_SPI_2_FS0  (via drill 0.33)
  Top 0.152: v28.7,13.11 28.7,12.83 28.02,12.14 27.46,12.14 27.02,12.58 U$3.53
  Bottom 0.152: U$3.53 27.02,12.58 27.46,12.14 28.02,12.14 28.7,12.83 v28.7,13.11
GP111_SPI_2_FS1  (via drill 0.33)
  Top 0.152: v27.74,12.8 27.56,12.98 U$3.51
  Bottom 0.152: U$3.51 27.56,12.98 v27.74,12.8
GP114_SPI_2_RXD  (via drill 0.33)
  Top 0.152: U$3.59 26.92,11.38 27.08,11.23 28.91,11.23 v29.03,11.35
  Bottom 0.152: U$3.59 26.92,11.38 27.08,11.23 28.91,11.23 v29.03,11.35
GP115_SPI_2_TXD  (via drill 0.33)
  Top 0.152: U$3.57 26.95,11.78 27.2,11.53 28.27,11.53 28.88,12.14 29.62,12.14 v29.64,12.17
  Bottom 0.152: U$3.57 26.95,11.78 27.2,11.53 28.27,11.53 28.88,12.14 29.62,12.14 v29.64,12.17
GP128_UART_1_CTS  (via drill 0.33)
  Top 0.152: U$3.65 26.9,10.18 27.84,9.25 v27.91,9.25
  Bottom 0.152: v27.91,9.25 27.84,9.25 26.9,10.18 U$3.65
GP129_UART_1_RTS  (via drill 0.33)
  Top 0.152: v28.93,10.34 28.5,9.91 27.66,9.91 26.99,10.58 U$3.63
  Bottom 0.152: U$3.63 26.99,10.58 27.66,9.91 28.5,9.91 v28.93,10.34
GP130_UART_1_RX  (via drill 0.33)
  Top 0.152: v27.94,10.57 27.61,10.9 26.95,10.9 26.87,10.98 U$3.61
  Bottom 0.152: U$3.61 26.87,10.98 26.95,10.9 27.61,10.9 v27.94,10.57
GP131_UART_1_TX  (via drill 0.33)
  Top 0.152: U$3.46 22.52,14.18 22.5,14.2 21.77,14.2 21.54,14.43 20.85,14.43 20.3,14.99 v20.07,14.99
  Bottom 0.152: v20.07,14.99 20.3,14.99 20.85,14.43 21.54,14.43 21.77,14.2 22.5,14.2 22.52,14.18 U$3.46
GP134_UART_2_RX  (via drill 0.33)
  Top 0.152: v21.77,18.95 21.8,18.98 U$3.22
  Bottom 0.152: U$3.22 21.8,18.98 v21.77,18.95
GP135_UART_2_TX  (via drill 0.33)
  Top 0.152: v29.39,18.54 29.06,18.54 28.73,18.21 28.35,18.21 27.76,17.63 27.23,17.63 27.08,17.78 U$3.27
  Bottom 0.152: U$3.27 27.08,17.78 27.23,17.63 27.76,17.63 28.35,18.21 28.73,18.21 29.06,18.54 v29.39,18.54
GP165  (via drill 0.33)
  Top 0.152: v27.48,18.29 27.38,18.18 U$3.25
  Bottom 0.152: U$3.25 27.38,18.18 v27.48,18.29
GP182_PWM2  (via drill 0.33)
  Top 0.152: U$3.37 27.02,15.78 27.1,15.7 27.61,15.7 28.14,16.23 v28.32,16.23
  Bottom 0.152: v28.32,16.23 28.14,16.23 27.61,15.7 27.1,15.7 27.02,15.78 U$3.37
GP183_PWM3  (via drill 0.33)
  Top 0.152: v29.39,16.41 29.39,16.36 28.6,15.57 27.91,15.57 27.74,15.39 26.62,15.39 26.61,15.38 U$3.39
  Bottom 0.152: U$3.39 26.61,15.38 26.62,15.39 27.74,15.39 27.91,15.57 28.6,15.57 29.39,16.36 v29.39,16.41
HV_SCL  (via drill 0.51)
  Top 0.254: U2.6 12.97,17.51 12.28,18.2 R2.1 12.28,19.9 v12.7,20.32 | U1.10 11.06,32.02 10.79,31.75 10.79,31.11 v11.18,30.73 | SJ4.2 14.42,25.72 v14.48,25.78
  Bottom 0.254: v11.18,30.73 11.81,30.1 11.81,27.05 12.19,26.67 12.7,26.67 13.08,26.29 13.08,25.91 13.21,25.78 v14.48,25.78 17.27,25.78 17.65,25.4 17.65,23.5 17.4,23.24 12.7,23.24 12.45,22.99 12.45,20.57 v12.7,20.32
HV_SDA  (via drill 0.51)
  Top 0.254: U2.5 13.47,17.15 14.39,18.07 R1.1 14.39,21.42 14.1,21.72 12.32,21.72 11.88,22.16 SJ3.2 11.88,25.47 v12.06,25.65 | v10.67,29.08 9.78,29.08 9.4,29.46 9.4,32.26 9.66,32.52 U1.9
  Bottom 0.254: v12.06,25.65 11.05,25.65 10.67,26.04 v10.67,29.08
MSIC_SLP_CLK  (via drill 0.33)
  Top 0.152: v27.51,21.46 27.19,21.78 U$3.7
  Bottom 0.152: U$3.7 27.19,21.78 v27.51,21.46
N$1
  Top 0.152: U2.7 12.47,17.25 12.32,17.4 12,17.4 11.97,17.37
  Top 0.254: U2.8 11.97,17.37 11.81,17.53 11.68,17.53 11.3,17.14 11.3,16.64 11.01,16.34 R3.1
N$3
  Top 0.254: R6.2 5.08,20.07 5.33,20.32 6.22,20.32 6.76,20.86 SJ1.2
OSC_CLK_OUT  (via drill 0.33)
  Top 0.152: v27.51,8.33 27.23,8.61 27.23,9.37 26.82,9.78 U$3.67
  Bottom 0.152: U$3.67 26.82,9.78 27.23,9.37 27.23,8.61 v27.51,8.33
PSW  (via drill 0.33)
  Top 0.152: v29.21,19.53 29.18,19.56 28.17,19.56 27.86,19.25 27.05,19.25 26.78,18.98 U$3.21
  Bottom 0.152: U$3.21 26.78,18.98 27.05,19.25 27.86,19.25 28.17,19.56 29.18,19.56 v29.21,19.53
PWRBTN#  (via drill 0.33)
  Top 0.152: v28.19,20.52 27.53,19.86 26.8,19.86 26.71,19.78 U$3.17
  Bottom 0.152: U$3.17 26.71,19.78 26.8,19.86 27.53,19.86 v28.19,20.52
RCVR_MODE  (via drill 0.33)
  Top 0.152: v28.65,17.55 28.12,17.55 27.89,17.32 26.92,17.32 26.58,16.98 U$3.31
  Bottom 0.152: U$3.31 26.58,16.98 26.92,17.32 27.89,17.32 28.12,17.55 v28.65,17.55
RESET_OUT#  (via drill 0.33)
  Top 0.152: U$3.36 22.25,16.18 21.82,15.75 20.5,15.75 v20.27,15.98
  Bottom 0.152: v20.27,15.98 20.5,15.75 21.82,15.75 22.25,16.18 U$3.36
USB_DN  (via drill 0.33)
  Top 0.152: U$3.18 22.61,19.78 22.48,19.91 19.61,19.91 18.97,20.55 v18.97,21.01
  Bottom 0.152: v18.97,21.01 18.97,20.55 19.61,19.91 22.48,19.91 22.61,19.78 U$3.18
USB_DP  (via drill 0.33)
  Top 0.152: U$3.16 22.67,20.18 22.5,20.34 20.12,20.34 v19.89,20.57
  Bottom 0.152: v19.89,20.57 20.12,20.34 22.5,20.34 22.67,20.18 U$3.16
USB_ID  (via drill 0.33)
  Top 0.152: v27.51,22.86 27.23,22.58 U$3.3
  Bottom 0.152: U$3.3 27.23,22.58 v27.51,22.86
USB_VBUS  (via drill 0.33)
  Top 0.152: v18.59,19.99 18.97,19.61 22.23,19.61 22.45,19.38 U$3.20
  Bottom 0.152: U$3.20 22.45,19.38 22.23,19.61 18.97,19.61 v18.59,19.99
V_BAT_BKUP  (via drill 0.33)
  Top 0.152: v28.45,18.87 28.37,18.95 27.18,18.95 26.81,18.58 U$3.23
  Bottom 0.152: U$3.23 26.81,18.58 27.18,18.95 28.37,18.95 v28.45,18.87
VSYS  (via drill 0.33, 0.51)
  Top 0.152: 22.35,22.61 22.35,22.35 22.52,22.18 22.86,22.18 | 22.35,22.61 22.35,22.86 22.47,22.98 | 22.47,22.98 | U$3.2 22.47,22.98 | U$3.6 22.86,22.18 | U$3.6 | U$3.6 22.86,22.18 | 22.86,22.18 | U$3.4 22.38,22.58 22.35,22.61
  Top 0.254: U1.8 12.95,33.02 13.12,32.85 C1.1 13.12,28.23 12.7,27.81 v9.53,27.81 | R1.2 16.09,21.93 16.51,22.35 v16.51,24.13 20.28,24.13 v21.19,23.22 | C2.1 7.62,15.49 7.87,15.24 R3.2 9.31,16.04 10.54,17.27 10.54,19.01 R2.2 10.58,21.17 9.34,22.41 SJ2.2 9.34,25.47 v9.53,25.65 | U$3.4 21.83,22.58 v21.19,23.22 | v21.19,23.22 v21.18,23.22
  Bottom 0.152: U$3.2 22.47,22.98 22.35,22.86 22.35,22.58 22.35,22.35 22.52,22.18 | U$3.6 22.52,22.18 | U$3.6 | U$3.6 22.52,22.18 | 22.52,22.18
  Bottom 0.254: v9.53,27.81 v9.53,25.65 9.53,24.51 9.91,24.13 v16.51,24.13 | v21.18,23.22 21.82,22.58 22.35,22.58 U$3.4

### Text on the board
Top: v10
tPlace: A1- / AIN3 | GND | A1+ / AIN2 | GND | A0- / AIN1 | GND | A0+ / AIN0 | GND | ADC Block | I2C ADDR / CLOSE ONE / ONLY | 0x48 | 0x49 | 0x4A | 0x4B
bPlace: A1- / AIN3 | GND | A1+ / AIN2 | GND | A0- / AIN1 | GND | A0+ / AIN0 | GND | ADC Block | 4xM2.0
tDocu: NOTE: Units are in Inches | M Hord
